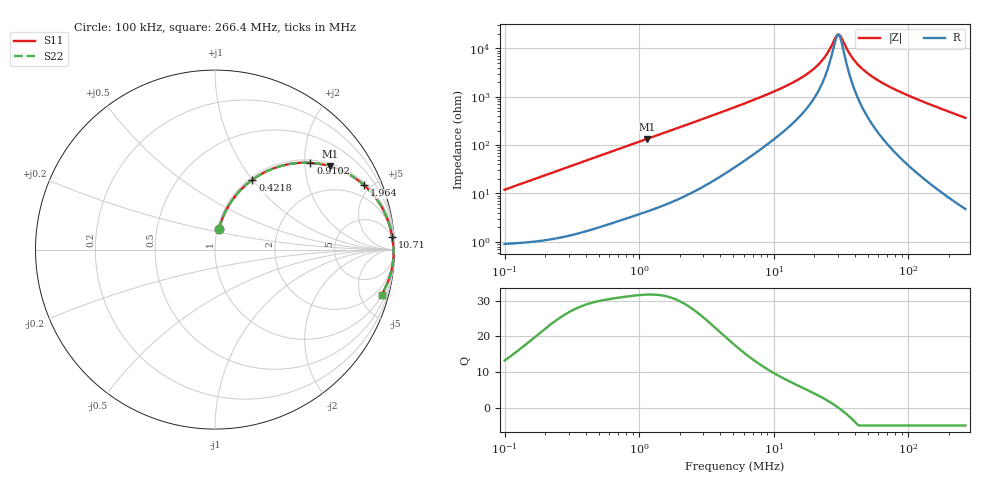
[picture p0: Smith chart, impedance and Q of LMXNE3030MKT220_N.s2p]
! LMXNE3030MKT220_N  S-PARAMETER MODEL  ( General Type )
! Model Generated by TAIYO YUDEN Corporation (http://www.ty-top.com)
! Version 1.0
! TAIYO YUDEN Control No. 191023NI43SB-FBB
! Copyright(c) 2019 TAIYO YUDEN CO.,LTD. All Rights Reserved.
! Product Description (link to TY-COMPAS)
! https://ds.yuden.co.jp/TYCOMPAS/or/detail?pn=LMXNE3030MKT220MN&u=M
! Products Name : Inductors
! Characteristics :
!  Inductance : 22 uH , SRF(min) : 22 MHz , DC Resistance(max) : 0.756 Ohm
!  Rated Current : Saturation :500 mA , Temp Rise : 500 mA
!  Case Size : 3.0 x 3.0 / 0.118 x 0.118 [mm/inch] , Thickness : 1.2 / 0.047 [mm/inch]
!  (Conditions: Temperature = 25 degC , DC Bias Current/Voltage = 0A / 0V)
! External Node Assignments :
!  1  o---GGG---o  2
! GND o---------o GND
! Frequency Range : 0.1MHz  -  266.375554MHz  [ 402 STEP ]
# MHz S RI R 50
! Freq[MHz].  S11 Real  S11 Imag  S21 Real  S21 Imag  S12 Real  S12 Imag  S22 Real  S22 Imag
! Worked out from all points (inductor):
!   401 points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, 100 kHz to 266.4 MHz, reference 50 ohm
!   read as one part in series: L = 19 uH near 104 kHz
!   highest Q = 31.7 at 1.153 MHz (marker M1), where L = 18.6 uH
!   self-resonance near 29.85 MHz
!   S11 on the Smith chart (normalised r, x): 100 kHz: 1.02, +0.24; 421.8 kHz: 1.03, +1.00; 910.2 kHz: 1.07, +2.13; 1.964 MHz: 1.15, +4.58; 10.71 MHz: 4, +28; 266.4 MHz: 1.10, -7.34
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0.1  0.0227 0.1157  0.9773 -0.1157  0.9773 -0.1157  0.0227 0.1157
0.211554  0.0688 0.2321  0.9312 -0.2321  0.9312 -0.2321  0.0688 0.2321
0.374775  0.1737 0.3616  0.8263 -0.3616  0.8263 -0.3616  0.1737 0.3616
0.421845  0.208 0.3891  0.792 -0.3891  0.792 -0.3891  0.208 0.3891
0.910203  0.5316 0.4833  0.4684 -0.4833  0.4684 -0.4833  0.5316 0.4833
1.153196  0.641 0.4642  0.359 -0.4642  0.359 -0.4642  0.641 0.4642
1.404561  0.7226 0.4321  0.2774 -0.4321  0.2774 -0.4321  0.7226 0.4321
1.963921  0.8318 0.3578  0.1682 -0.3578  0.1682 -0.3578  0.8318 0.3578
5.26394  0.9666 0.1529  0.0334 -0.1529  0.0334 -0.1529  0.9666 0.1529
10.70546  0.9872 0.0702  0.0128 -0.0702  0.0128 -0.0702  0.9872 0.0702
14.96887  0.991 0.044  0.00902 -0.044  0.00902 -0.044  0.991 0.044
19.34272  0.9929 0.027  0.00711 -0.027  0.00711 -0.027  0.9929 0.027
23.55889  0.994 0.0149  0.00603 -0.0149  0.00603 -0.0149  0.994 0.0149
28.69407  0.9947 0.00308  0.00526 -0.00308  0.00526 -0.00308  0.9947 0.00308
30.44272  0.9949 -0.000468  0.00509 0.000468  0.00509 0.000468  0.9949 -0.000468
31.66729  0.995 -0.00284  0.005 0.00284  0.005 0.00284  0.995 -0.00284
37.81678  0.9952 -0.0137  0.00475 0.0137  0.00475 0.0137  0.9952 -0.0137
43.41409  0.9952 -0.0226  0.00479 0.0226  0.00479 0.0226  0.9952 -0.0226
53.93017  0.9947 -0.0375  0.00532 0.0375  0.00532 0.0375  0.9947 -0.0375
72.49162  0.9927 -0.0609  0.00731 0.0609  0.00731 0.0609  0.9927 -0.0609
128.421  0.9814 -0.1227  0.0186 0.1227  0.0186 0.1227  0.9814 -0.1227
266.3756  0.9281 -0.2519  0.0719 0.2519  0.0719 0.2519  0.9281 -0.2519
